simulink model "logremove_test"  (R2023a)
settings: Solver=FixedStepDiscrete  StartTime=0.0  StopTime=10  FixedStep=1  RelTol=1e-3
libraries: simulink x1

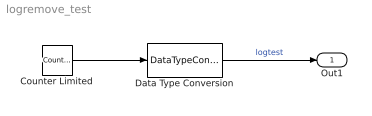
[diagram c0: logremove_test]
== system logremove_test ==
  Counter Limited : simulink/Sources/Counter Limited  uplimit=7  tsamp=-1
  Data Type Conversion : DataTypeConversion
  Out1 : Outport  VectorParamsAs1DForOutWhenUnconnected=off
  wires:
  Counter Limited/1 -> Data Type Conversion/1
  Data Type Conversion/1 -> Out1/1  "logtest"
